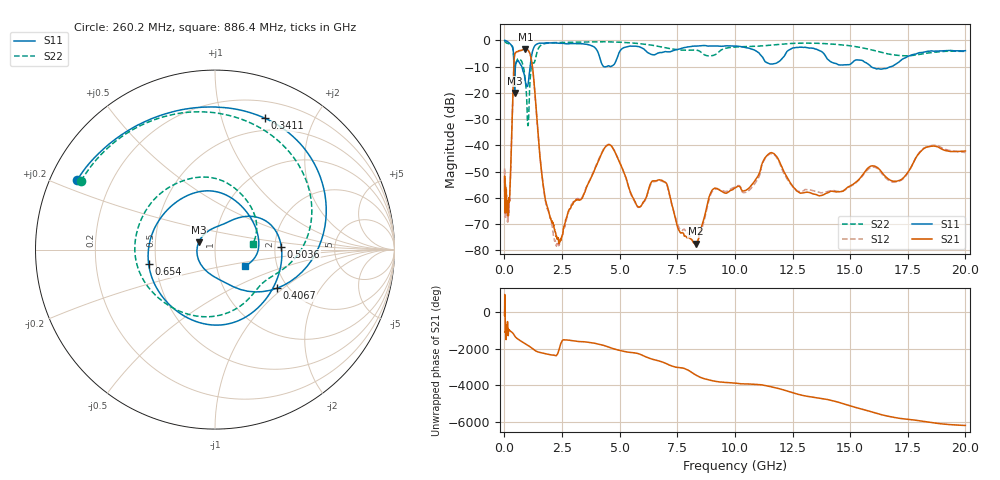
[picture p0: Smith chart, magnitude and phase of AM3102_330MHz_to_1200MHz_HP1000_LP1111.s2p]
! Date/Time: Tue, Sep 11, 2018 5:17 PM
! Network Analyzer: Agilent Technologies E8362B Rev: A.07.50.63
! Sweep from 0.010 to 20.000 GHz, 1601 Points, Sweep Type: LOG
! Power Supply: 4.949 V, 0.001 A
# Hz S DB R 50
!freq MagS11 AngS11 MagS21 AngS21 MagS12 AngS12 MagS22 AngS22
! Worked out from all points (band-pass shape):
!   1601 points, 10 MHz to 20 GHz, reference 50 ohm
!   highest |S21| = -3.21 dB at 916.3 MHz (marker M1); lowest = -77.5 dB at 8.305 GHz (marker M2)
!   |S21| within 3 dB of the highest: 432.6 MHz to 1.145 GHz (712.8 MHz wide, 90.3 % of centre)
!   lowest |S11| = -20.0 dB at 440.9 MHz (marker M3), VSWR 1.22, Z = 41.5 + j3.34 ohm
!   |S11| at or under -10 dB: 413.1 MHz to 478.1 MHz (65.05 MHz wide, 14.6 % of centre); 759.2 MHz to 1.116 GHz (356.5 MHz wide, 38 % of centre); 15.91 GHz to 16.76 GHz (852.1 MHz wide, 5.22 % of centre)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
!   |S22| runs from -32.5 to -0.2 dB; largest |S21 - S12| = 0.0093
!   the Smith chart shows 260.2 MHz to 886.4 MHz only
!   S11 on the Smith chart (normalised r, x): 260.2 MHz: 0.08, +0.24; 341.1 MHz: 0.37, +1.39; 406.7 MHz: 1.76, -0.91; 503.6 MHz: 2.17, +0.08; 654 MHz: 0.46, -0.09; 886.4 MHz: 1.38, -0.26
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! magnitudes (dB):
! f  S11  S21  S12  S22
! 10 MHz  0.0  -59.4  -54.0  -0.2
! 35.55 MHz  0.0  -59.9  -64.6  -0.5
! 126.4 MHz  -0.4  -64.0  -64.8  -1.1
! 260.2 MHz  -1.3  -52.8  -53.5  -1.5
! 341.1 MHz  -2.1  -29.0  -29.0  -2.4
! 406.7 MHz  -7.8  -10.1  -10.1  -6.1
! 440.9 MHz  -20.0  -5.6  -5.7  -9.7
! 447.2 MHz  -19.4  -5.3  -5.4  -9.9
! 503.6 MHz  -8.6  -4.5  -4.5  -8.4
! 654 MHz  -8.4  -3.9  -4.0  -7.1
! 886.4 MHz  -14.3  -3.3  -3.3  -13.4
! 916.3 MHz  -15.9  -3.2  -3.3  -15.8
! 1.027 GHz  -16.8  -3.7  -3.8  -32.4
! 1.59 GHz  -1.1  -48.2  -48.2  -1.8
! 2.314 GHz  -1.0  -75.7  -77.6  -0.8
! 4.457 GHz  -9.9  -40.0  -39.8  -0.5
! 5.652 GHz  -2.2  -61.2  -61.4  -1.0
! 6.835 GHz  -4.6  -53.3  -53.6  -2.5
! 8.305 GHz  -2.1  -77.5  -77.5  -3.7
! 11.53 GHz  -9.0  -42.9  -43.2  -1.8
! 13.81 GHz  -4.5  -58.9  -58.0  -1.2
! 20 GHz  -3.9  -42.1  -42.7  -4.2
